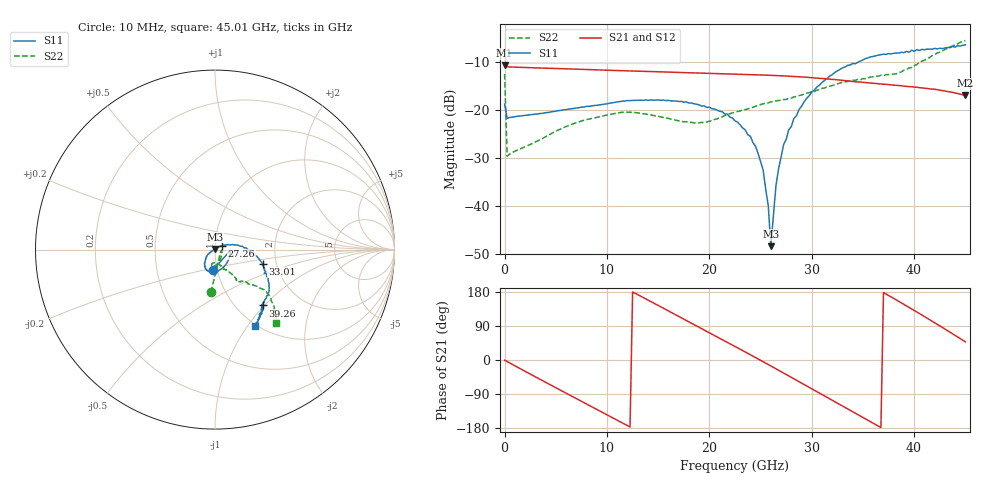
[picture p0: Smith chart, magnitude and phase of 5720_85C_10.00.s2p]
! Device:  ADRF5720
! Description: 0.5dB LSB GaAs MMIC 6-bit Digital Attenuator
! Frequency:  0.000009 -  40 GHz
! Ports:
!	RF1	= Port 1
!	RF2	= Port 2
! Vdd:  3.3 Volt
! Vss:  -3.3 Volt
! Control:  0/3.3 Volt
! State:  10.00 dB attenuation
! Data:  The device was measured using G-S-G Probes on a matrix board.
!  Data was collected using an calibrated 4 port network analyzer.
!  The reference plane for this measurement is at the launchers.
! Note:  Analog Devices supplies this data as a sample of measured data
!  for this product.  Your particular data for this product may vary.
!  Data was taken at 85 degrees C.
!  Analog Devices reserves the right to change this data at anytime.
# GHZ S DB R 45.0
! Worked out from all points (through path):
!   181 points, 10 MHz to 45.01 GHz, reference 45 ohm
!   highest |S21| = -10.68 dB at 10 MHz (marker M1); lowest = -16.9 dB at 45.01 GHz (marker M2)
!   group delay of S21, straight-line fit = 41 ps
!   lowest |S11| = -48.4 dB at 26.01 GHz (marker M3), VSWR 1.01, Z = 44.9 + j0.337 ohm
!   |S11| at or under -10 dB: start of sweep to 34.53 GHz
!   |S22| runs from -29.6 to -5.5 dB; largest |S21 - S12| = 0.0014
!   S11 on the Smith chart (normalised r, x): 10 MHz: 0.95, -0.22; 27.26 GHz: 1.08, +0.04; 33.01 GHz: 1.69, -0.29; 39.26 GHz: 1.32, -0.98; 45.01 GHz: 0.98, -1.08
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0.01  -18.74 -96.6  -10.68 -0.7  -10.66 -0.6  -12.44 -95.5
0.26  -21.70 -7.3  -10.97 -4.0  -10.97 -4.0  -29.60 -14.3
4.26  -20.48 -38.5  -11.26 -62.4  -11.25 -62.4  -25.25 -51.8
7.76  -19.33 -63.1  -11.50 -112.6  -11.49 -112.5  -22.11 -75.9
11.51  -18.12 -85.3  -11.77 -166.1  -11.76 -165.9  -20.44 -94.5
15.26  -17.93 -104.0  -12.00 140.3  -12.00 140.5  -21.41 -103.1
19.01  -18.90 -118.8  -12.25 86.5  -12.25 86.7  -22.66 -87.5
22.76  -22.48 -133.2  -12.51 32.2  -12.50 32.4  -20.26 -69.8
24.01  -25.45 -143.4  -12.59 13.9  -12.58 14.1  -19.60 -67.8
24.51  -27.51 -144.5  -12.63 6.6  -12.62 6.8  -19.18 -67.6
25.26  -32.49 -157.7  -12.67 -4.5  -12.67 -4.2  -18.70 -66.0
25.76  -39.95 -172.0  -12.71 -11.9  -12.71 -11.7  -18.49 -65.1
26.01  -48.36 101.2  -12.73 -15.7  -12.72 -15.4  -18.26 -64.6
26.51  -35.74 44.5  -12.77 -23.2  -12.77 -22.9  -18.04 -63.1
27.26  -27.15 27.2  -12.85 -34.5  -12.85 -34.2  -17.79 -61.7
28.26  -21.72 19.3  -12.98 -49.5  -12.97 -49.2  -17.23 -59.9
30.26  -15.81 3.5  -13.27 -79.8  -13.26 -79.5  -16.11 -56.5
33.01  -11.17 -16.5  -13.78 -121.6  -13.77 -121.3  -14.18 -54.5
37.76  -8.27 -41.8  -14.73 166.3  -14.72 166.6  -12.46 -48.0
39.26  -7.73 -49.2  -15.04 142.8  -15.03 143.2  -11.56 -46.1
42.26  -7.23 -54.8  -15.72 94.2  -15.70 94.7  -8.07 -40.2
45.01  -6.36 -62.6  -16.92 47.9  -16.90 48.4  -5.46 -50.2
